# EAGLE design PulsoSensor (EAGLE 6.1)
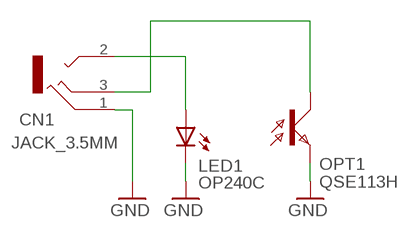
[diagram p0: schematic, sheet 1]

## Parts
CN1  JACK_3.5MM  [JACK_3.5MM]
LED1  OP240C  LEDV  [LATERAL_V]
OPT1  QSE113H  [LATERAL_H]

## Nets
GND: CN1.1 LED1.E(C) OPT1.E
N$1: CN1.3 OPT1.C
N$2: CN1.2 LED1.C(A)

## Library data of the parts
CN1 = 00-LIVIO:JACK_3.5MM
LED1 = 00-LIVIO:LED: LEDS
OPT1 = 00-LIVIO:QSE113: PHOTO TRANSISTOR

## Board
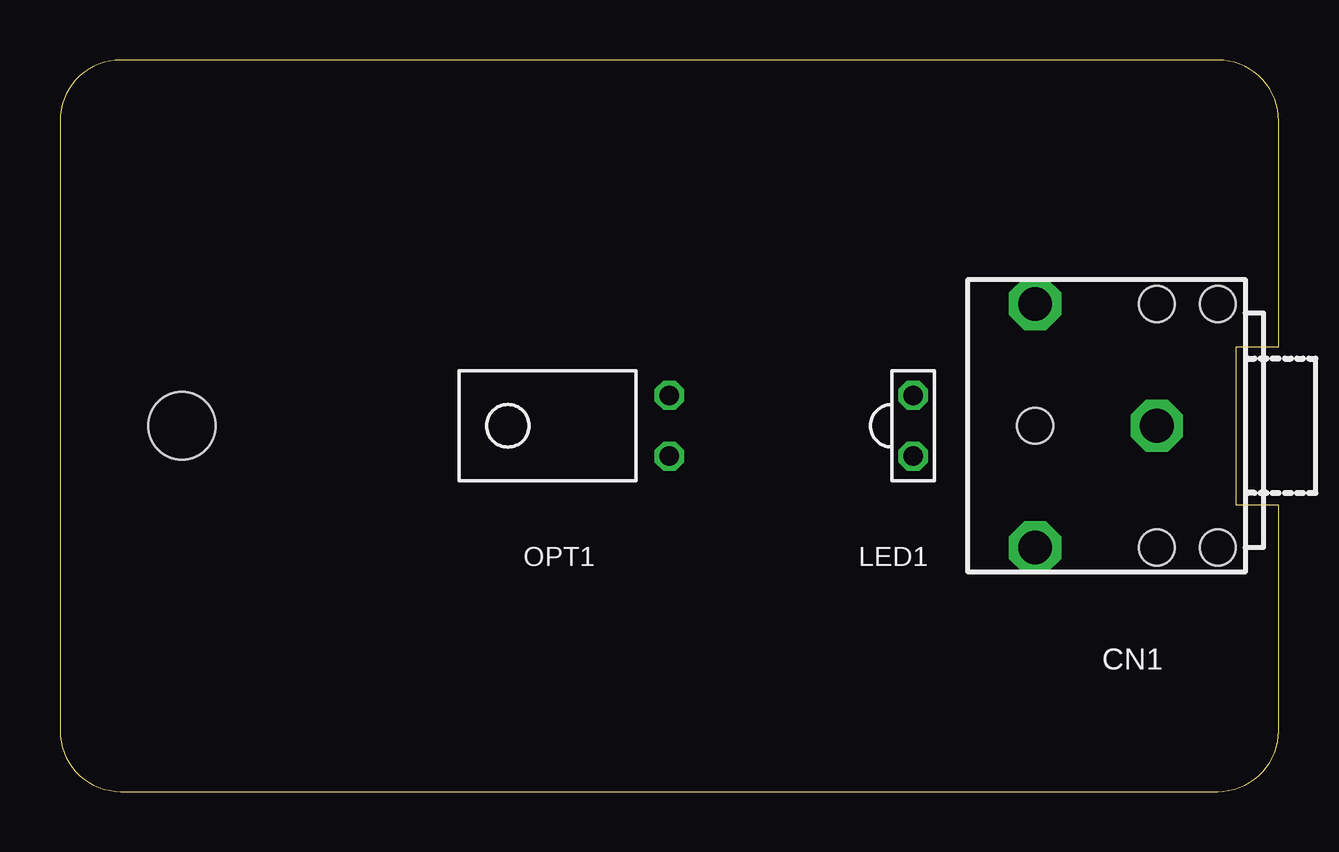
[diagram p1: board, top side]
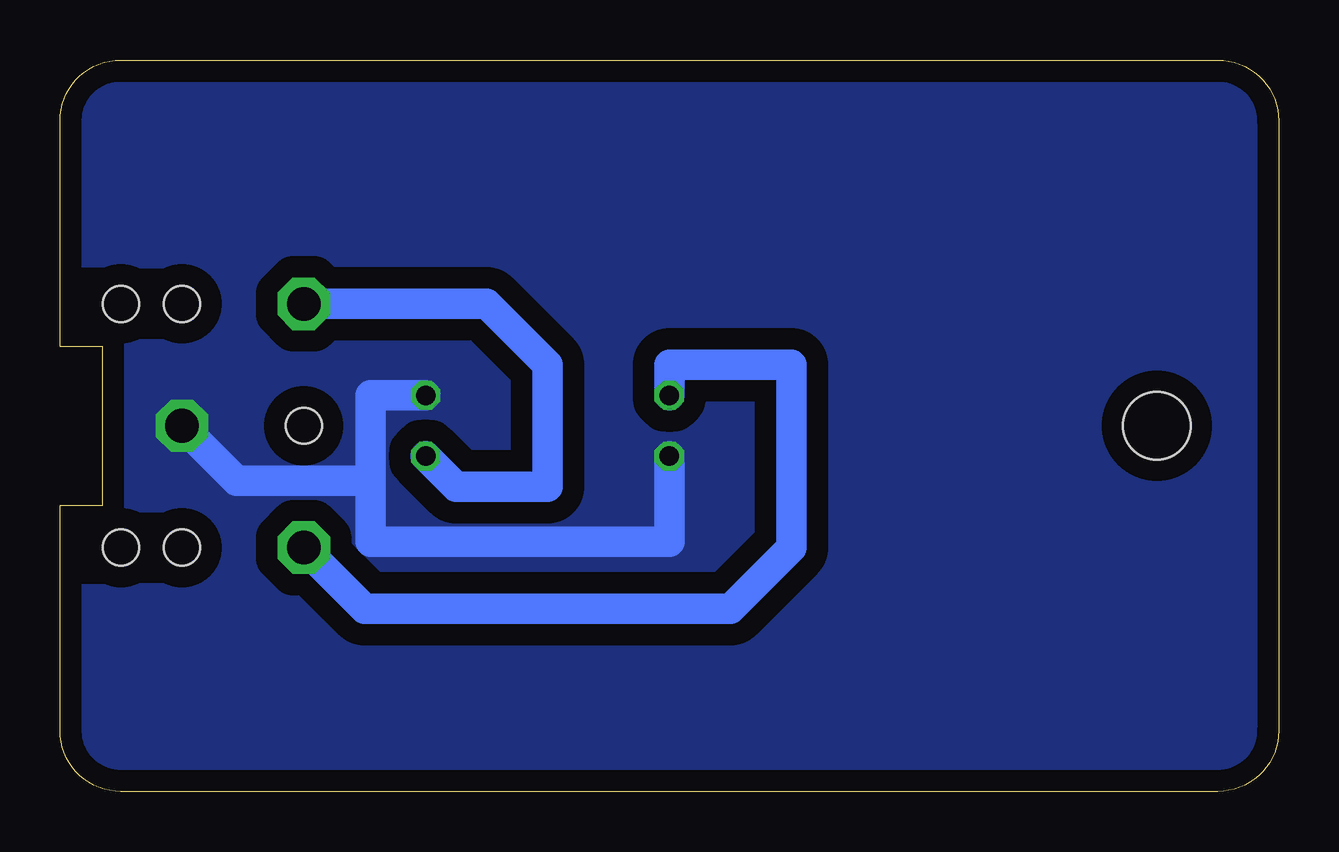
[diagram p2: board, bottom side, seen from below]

Size 50.8 x 30.48 mm. Coordinates in mm from the lower left corner, seen from the top.
Outline: 0,27.94 0,2.54 arc90 2.54,0 48.26,0 arc90 50.8,2.54 50.8,11.94 49.02,11.94 49.02,18.54 50.8,18.54 50.8,27.94 arc90 48.26,30.48 2.54,30.48 arc90 0,27.94
Copper layers (1*16): Top 0.035mm / dielectric 1.5mm / Bottom 0.035mm
Design rules: minimum track width 10mil, minimum drill 31mil, track to track 31mil, track to pad 31mil, pad to pad 31mil, via to via 31mil, smd to smd 31mil, copper to edge 31mil, drill to drill 8mil, minimum pad ring 5mil, minimum via ring 8mil, stop-mask expansion 4mil, vias tented up to drill 0mil, thermal gap 47mil
Holes 2.8 mm at 5.08,15.24

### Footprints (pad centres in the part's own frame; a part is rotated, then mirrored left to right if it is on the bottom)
JACK_3.5MM = drill 1.4 pad 2.184 octagon: 1 0,0; 2 -5.08,-5.08; 3 5.08,-5.08 | hole 1.5: -5.08,0; -5.08,2.54; 5.08,0; 5.08,2.54; 0,-5.08
LATERAL_V = drill 0.813 octagon: C 0,-1.27; E 0,1.27
LATERAL_H = drill 0.813 octagon: C 0,-1.27; E 0,1.27

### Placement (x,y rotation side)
CN1  45.72,15.24 270 top
LED1  35.56,15.24 0 top
OPT1  25.4,15.24 180 top

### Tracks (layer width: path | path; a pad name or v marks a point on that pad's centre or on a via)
GND
  Bottom 1.27: LED1.E 37.85,16.51 37.85,15.24 37.85,13.21 | 37.85,13.21 38.1,12.95 43.43,12.95 CN1.1 | OPT1.E 25.4,10.41 37.85,10.41 37.85,13.21
  pour Bottom (isolate 0.9, rank 6, no thermals): -1,31.48 -1,-1 51.8,-1 51.8,31.48
N$1
  Bottom 1.27: OPT1.C 25.4,17.78 20.32,17.78 20.32,10.16 22.86,7.62 38.1,7.62 CN1.3
N$2
  Bottom 1.27: LED1.C 34.29,12.7 30.48,12.7 30.48,17.78 33.02,20.32 CN1.2

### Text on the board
tValues: Theremino PulsoSensor V2 | 30 x 50 mm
